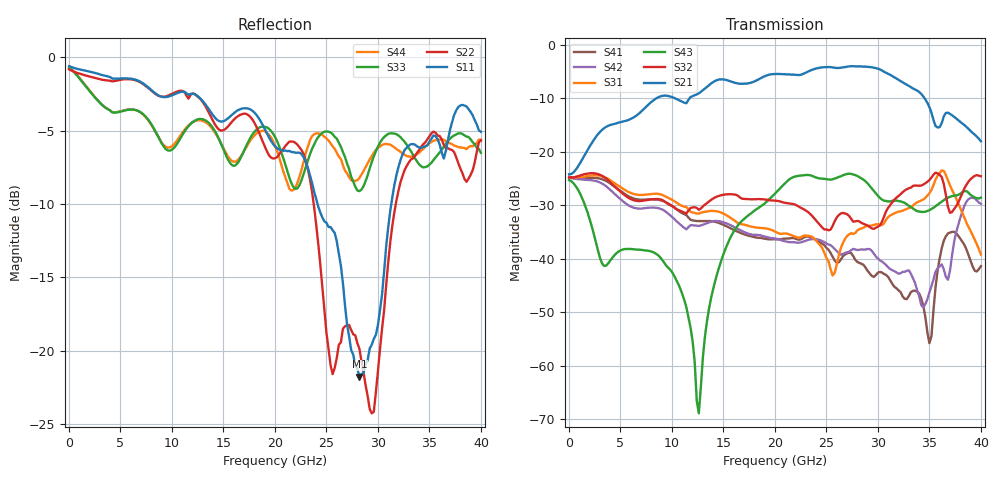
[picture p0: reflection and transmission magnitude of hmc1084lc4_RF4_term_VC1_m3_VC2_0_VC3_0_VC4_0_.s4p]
!Agilent Technologies,N5224A,MY51441122,A.09.40.06
!Agilent N5224A: A.09.40.06
!Date: Thursday, June 19, 2014 00:54:04
!Correction: S11(Full 4 Port(1,2,3,4))
!S12(Full 4 Port(1,2,3,4))
!S13(Full 4 Port(1,2,3,4))
!S14(Full 4 Port(1,2,3,4))
!S21(Full 4 Port(1,2,3,4))
!S22(Full 4 Port(1,2,3,4))
!S23(Full 4 Port(1,2,3,4))
!S24(Full 4 Port(1,2,3,4))
!S31(Full 4 Port(1,2,3,4))
!S32(Full 4 Port(1,2,3,4))
!S33(Full 4 Port(1,2,3,4))
!S34(Full 4 Port(1,2,3,4))
!S41(Full 4 Port(1,2,3,4))
!S42(Full 4 Port(1,2,3,4))
!S43(Full 4 Port(1,2,3,4))
!S44(Full 4 Port(1,2,3,4))
!S4P File: Measurements: <S11,S12,S13,S14>,
!<S21,S22,S23,S24>,
!<S31,S32,S33,S34>,
!<S41,S42,S43,S44>:
# Hz S  dB  R 50
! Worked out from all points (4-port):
!   201 points, 10 MHz to 40 GHz, reference 50 ohm
!   strongest paths, dB at 10 MHz, 10.01 GHz, 20 GHz, 30 GHz, 40 GHz:
!     S21: -24.2, -9.8, -5.4, -4.4, -18.0
!     S32: -24.8, -30.1, -29.1, -34.0, -24.6
!     S43: -25.3, -42.5, -27.8, -28.2, -28.6
!     S31: -24.8, -29.0, -34.9, -33.5, -39.2
!     S42: -24.8, -32.2, -36.2, -40.0, -29.7
!     S41: -24.7, -30.1, -36.4, -42.6, -41.4
!   lowest |S11| = -21.8 dB at 28.2 GHz (marker M1), VSWR 1.18, Z = 55.7 - j6.49 ohm
!   |S11| at or under -10 dB: 24.13 GHz to 31.3 GHz (7.167 GHz wide, 25.9 % of centre)
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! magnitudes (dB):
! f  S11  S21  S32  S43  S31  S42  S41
! 10 MHz  -0.6  -24.2  -24.8  -25.3  -24.8  -24.8  -24.7
! 10.21 GHz  -2.5  -9.9  -30.3  -43.2  -29.2  -32.5  -30.4
! 12.61 GHz  -2.7  -9.0  -30.9  -68.9  -31.6  -33.9  -33.0
! 16.21 GHz  -3.7  -7.1  -28.0  -34.3  -33.1  -34.2  -34.8
! 28.2 GHz  -21.8  -4.0  -33.0  -24.7  -34.5  -38.3  -40.8
! 34.4 GHz  -6.1  -9.6  -26.1  -31.3  -28.9  -49.1  -48.8
! 40 GHz  -5.1  -18.0  -24.6  -28.6  -39.2  -29.7  -41.4
